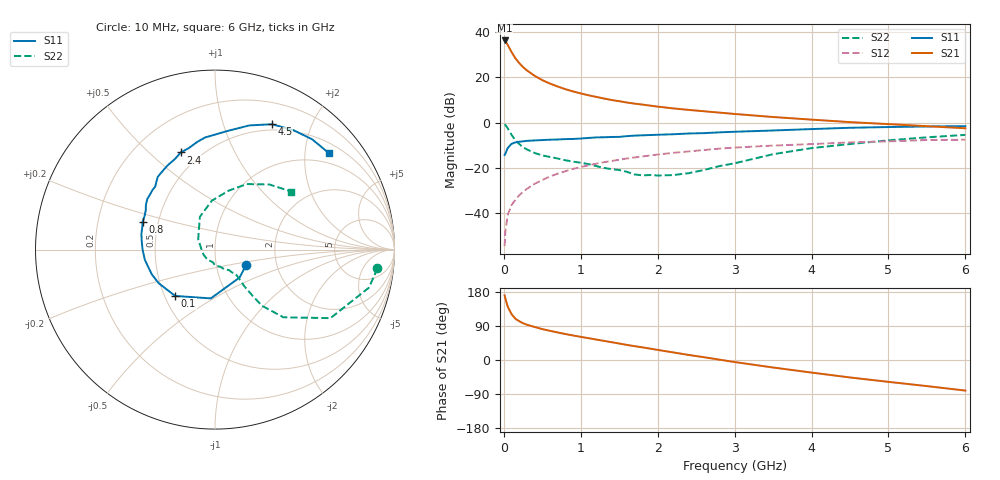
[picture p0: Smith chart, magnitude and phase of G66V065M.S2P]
! SIEMENS Small Signal Semiconductors
! BFG193
! Si NPN RF Bipolar Junction Transistor in SOT223
! VCE = 6 V  IC = 65 mA
! Common Emitter S-Parameters:  August  1996
# GHz  S  MA  R  50
!  f  S11  S21  S12  S22
! GHz  MAG  ANG  MAG  ANG  MAG  ANG  MAG  ANG
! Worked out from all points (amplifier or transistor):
!   36 points, 10 MHz to 6 GHz, reference 50 ohm
!   highest |S21| = 36.1 dB at 10 MHz (marker M1)
!   |S21| within 3 dB of that: start of sweep to 66.91 MHz
!   unconditionally stable (mu >= 1): 407.3 MHz to 2.395 GHz
!   at 250 MHz: K = 0.94, MSG = 27.5 dB, |S12| = -30.6 dB
!   at 1.4 GHz: K = 1.04, MAG = 12.1 dB, |S12| = -16.9 dB
!   at 6 GHz: K = 0.89, MSG = 2.5 dB, |S12| = -7.6 dB
!   S11 on the Smith chart (normalised r, x): 10 MHz: 1.40, -0.25; 100 MHz: 0.57, -0.33; 800 MHz: 0.41, +0.16; 2.4 GHz: 0.39, +0.63; 4.5 GHz: 0.43, +1.46; 6 GHz: 0.73, +2.55
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0.01  0.1939 -25.8  64.07 170.4  0.0019 85.3  0.9112 -6.6
0.02  0.2073 -48.7  61.71 162.4  0.004 80.5  0.8833 -13.9
0.05  0.273 -94.9  51.29 140.9  0.0092 71.6  0.7481 -30.7
0.1  0.3405 -130.7  35.67 121.1  0.0153 67.9  0.5362 -44.7
0.15  0.3654 -149.2  25.99 108.9  0.0198 67.5  0.4079 -50.1
0.2  0.378 -158.5  20.38 102.3  0.0251 69.7  0.337 -50.8
0.25  0.3862 -166.7  16.61 97.0  0.0296 70.0  0.2853 -51.2
0.3  0.395 -171.7  14.03 93.1  0.0348 70.3  0.2563 -51.3
0.4  0.4036 179.8  10.68 87.1  0.0448 70.4  0.2137 -50.4
0.5  0.4111 173.3  8.572 81.5  0.0545 69.4  0.1893 -49.8
0.6  0.419 168.2  7.202 77.0  0.0649 68.6  0.1749 -50.6
0.8  0.4319 158.8  5.42 68.5  0.0847 65.0  0.1479 -54.6
0.9  0.435 154.3  4.835 64.7  0.0957 63.5  0.138 -55.7
1.1  0.4581 147.2  3.98 57.6  0.1145 59.9  0.1217 -64.7
1.3  0.4739 140.1  3.38 50.5  0.1338 55.7  0.1005 -72.3
1.6  0.502 130.4  2.756 39.8  0.1619 49.0  0.0823 -92.7
2.2  0.5521 113.8  2.048 20.1  0.2152 35.3  0.0698 -155.9
2.4  0.5739 109.4  1.899 13.4  0.2313 31.1  0.0767 176.3
3.5  0.6683 83.2  1.323 -19.8  0.3111 4.1  0.201 114.8
4.5  0.7669 65.6  1.021 -46.1  0.366 -16.1  0.3363 77.1
5.5  0.819 48.6  0.831 -68.9  0.412 -39.4  0.4728 50.1
6  0.8319 40.2  0.748 -80.7  0.4181 -52.9  0.5347 37.2
